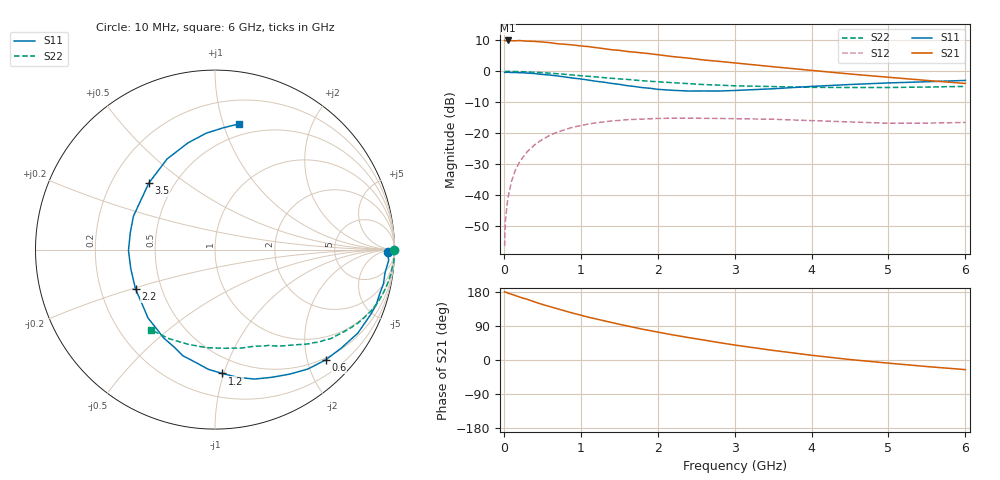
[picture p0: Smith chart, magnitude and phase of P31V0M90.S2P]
! SIEMENS Small Signal Semiconductors
! BFP181
! Si NPN RF Bipolar Junction Transistor in SOT143
! VCE = 1 V  IC = 0.9 mA
! Common Emitter S-Parameters:  March  1996
# GHz  S  MA  R  50
!  f  S11  S21  S12  S22
! GHz  MAG  ANG  MAG  ANG  MAG  ANG  MAG  ANG
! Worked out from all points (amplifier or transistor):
!   36 points, 10 MHz to 6 GHz, reference 50 ohm
!   highest |S21| = 10.0 dB at 50 MHz (marker M1)
!   |S21| within 3 dB of that: start of sweep to 1.402 GHz
!   unconditionally stable (mu >= 1): 3 GHz to end of sweep
!   at 250 MHz: K = 0.10, MSG = 18.8 dB, |S12| = -27.7 dB
!   at 1.4 GHz: K = 0.51, MSG = 11.5 dB, |S12| = -16.0 dB
!   at 6 GHz: K = 1.39, MAG = 2.6 dB, |S12| = -16.5 dB
!   S11 on the Smith chart (normalised r, x): 10 MHz: 45, -19; 600 MHz: 0.46, -2.34; 1.2 GHz: 0.37, -0.99; 2.2 GHz: 0.35, -0.21; 3.5 GHz: 0.36, +0.37; 6 GHz: 0.40, +1.13
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0.01  0.963 -0.9  3.155 179.7  0.0015 89.1  0.9983 -0.2
0.02  0.9623 -1.6  3.117 179.4  0.0038 89.1  0.9927 -0.7
0.05  0.9697 -3.5  3.157 176.7  0.0085 89.2  0.9974 -1.9
0.1  0.9559 -7.8  3.127 173.5  0.0169 83.9  0.9986 -3.7
0.2  0.9496 -15.4  3.147 166.5  0.0336 79.8  0.9906 -7.4
0.4  0.9219 -30.3  3.049 153.3  0.065 69.9  0.9677 -14.6
0.5  0.8923 -37.9  2.98 146.7  0.0794 64.8  0.9527 -18.1
0.6  0.8704 -44.9  2.909 140.8  0.093 60.0  0.9343 -21.4
0.9  0.7791 -65.9  2.669 123.5  0.1252 47.3  0.8732 -29.9
1.1  0.7228 -80.0  2.512 112.9  0.1411 39.9  0.8306 -35.1
1.2  0.6914 -86.6  2.414 108.3  0.1476 36.1  0.8134 -37.6
1.5  0.6178 -106.9  2.186 94.3  0.1612 27.7  0.755 -43.4
1.8  0.5457 -127.4  1.983 81.3  0.1696 20.6  0.7062 -48.5
2.2  0.494 -153.7  1.729 66.1  0.1753 12.2  0.6556 -54.9
2.4  0.4812 -167.2  1.636 59.2  0.1753 8.5  0.6334 -58.0
2.8  0.4814 168.5  1.449 45.9  0.1736 2.9  0.5997 -63.8
3  0.4911 157.7  1.37 39.5  0.1719 0.0  0.584 -66.9
3.5  0.5232 134.7  1.188 25.3  0.1684 -4.5  0.5679 -74.9
4  0.5714 117.8  1.037 12.5  0.1602 -7.8  0.5523 -84.5
4.5  0.6134 104.2  0.907 1.2  0.1524 -10.0  0.5485 -95.2
5.5  0.6797 86.2  0.713 -17.3  0.1458 -7.5  0.5584 -117.3
6  0.714 79.0  0.638 -25.4  0.1496 -6.1  0.5713 -128.6
